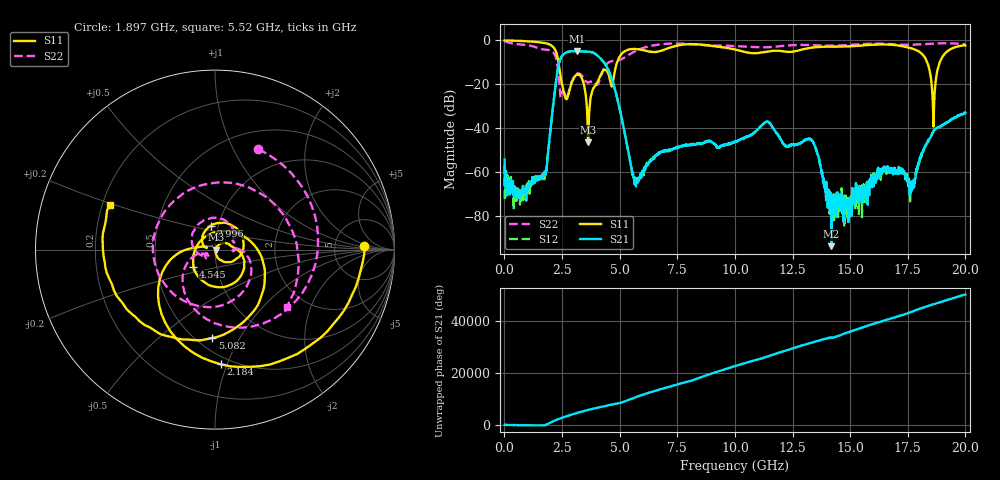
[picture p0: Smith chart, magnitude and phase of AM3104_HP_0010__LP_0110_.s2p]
!Created with skrf (http://scikit-rf.org).
# Hz S RI R 50.0
!freq ReS11 ImS11 ReS21 ImS21 ReS12 ImS12 ReS22 ImS22
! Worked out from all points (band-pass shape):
!   1601 points, 10 MHz to 20 GHz, reference 50 ohm
!   highest |S21| = -4.79 dB at 3.146 GHz (marker M1); lowest = -93.8 dB at 14.19 GHz (marker M2)
!   |S21| within 3 dB of the highest: 2.459 GHz to 4.129 GHz (1.67 GHz wide, 50.7 % of centre)
!   lowest |S11| = -46.5 dB at 3.633 GHz (marker M3), VSWR 1.01, Z = 50.5 - j0.122 ohm
!   |S11| at or under -10 dB: 2.348 GHz to 4.89 GHz (2.542 GHz wide, 70.2 % of centre); 18.34 GHz to 18.89 GHz (541.9 MHz wide, 2.91 % of centre)
!   |S22| runs from -26.3 to -0.2 dB; largest |S21 - S12| = 0.0053
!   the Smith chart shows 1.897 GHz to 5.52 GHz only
!   S11 on the Smith chart (normalised r, x): 1.897 GHz: 11, +2; 2.184 GHz: 0.44, -0.95; 2.996 GHz: 0.92, +0.25; 4.545 GHz: 0.77, -0.15; 5.082 GHz: 0.59, -0.77; 5.52 GHz: 0.23, +0.19
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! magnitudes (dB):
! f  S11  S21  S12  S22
! 10 MHz  0.0  -54.3  -56.9  -0.2
! 759.6 MHz  -0.2  -69.8  -70.2  -1.8
! 1.897 GHz  -1.6  -51.0  -51.1  -4.3
! 2.184 GHz  -3.9  -23.5  -23.5  -6.4
! 2.646 GHz  -26.0  -5.6  -5.6  -25.2
! 2.996 GHz  -17.4  -4.8  -4.8  -17.0
! 3.146 GHz  -15.6  -4.8  -4.8  -15.1
! 3.346 GHz  -16.8  -5.0  -5.0  -15.8
! 3.633 GHz  -46.5  -5.2  -5.2  -19.1
! 4.545 GHz  -16.3  -14.3  -14.3  -9.8
! 5.082 GHz  -6.2  -35.1  -35.0  -8.5
! 5.52 GHz  -3.9  -58.8  -58.7  -5.8
! 6.682 GHz  -5.1  -51.7  -51.3  -1.9
! 10.01 GHz  -4.1  -46.3  -46.2  -2.6
! 11.39 GHz  -5.1  -37.0  -37.0  -3.0
! 13.34 GHz  -3.2  -45.6  -45.5  -2.2
! 14.19 GHz  -2.8  -93.8  -76.1  -2.3
! 16.68 GHz  -1.9  -59.7  -58.2  -1.6
! 17.7 GHz  -3.8  -66.3  -65.4  -1.9
! 18.61 GHz  -39.3  -41.5  -41.3  -1.4
! 19.03 GHz  -7.1  -38.4  -38.5  -1.3
! 20 GHz  -2.2  -33.0  -32.9  -1.7
